FUNCTION_BLOCK FB_IEDServerSession IMPLEMENTS I_ScsmAbortIndEventSink, I_ScsmAssociateIndEventSink, I_ScsmReleaseIndEventSink
VAR_INPUT
	fbConnection		: FB_iec61850ConnectionClass := (ipAbortInd:=THIS^, ipAssociateInd:=THIS^, ipReleaseInd:=THIS^);
END_VAR
VAR
	_bAbort				: BOOL; (* Rising edge activates AbortReq() command execution *)
	_bDisconnect		: BOOL; (* Rising edge activates ReleaseReq() command execution *)
	
	state				: BYTE;
	eState				: E_AsyncEnvironmentState; (* Environment state *)
	bBusy				: BOOL; (* If TRUE => command execution is busy *)
	bSuccess			: BOOL;
	ipResult			: I_AsyncServiceResultClass;
	sLastErrorResult	: T_MaxString;
	fbAbortReason		: FB_ServiceErrorClass := (stError:=SUCCESS_EVENT);
	sLastAbortReason	: T_MaxString;
END_VAR

fbConnection.Execute();
eState:= fbConnection.eState;

(* Execute server control block implementations *)
fbIED.IEDLD1.LLN0.urcb101.Server.Execute();
fbIED.IEDLD1.LLN0.brcb101.Server.Execute();

(* 
	a) The unbuffered report control block IEDLD1/LLN0.urcb101 requires time stamp values in BinaryTime format. 
	We use the unbuffered reporting to test our user defined clock implementation.
	The internal unbuffered report control block implementation queries our user defined clock for new time stamp value.
	
	b) The attribute IEDLD1/MMXU1.TotW.t requires time stamp value in UtcTime format.
	Read of the attribute "IEDLD1/MMXU1.TotW" or "IEDLD1/MMXU1.TotW.t" (e.g. GetDataValues service) triggers the execution IEDLD1/MMXU1.TotW.OnGetVPreEvent() method and 
	queries our user defined clock for new time stamp value.
*)

CASE state OF
	0: (* Initial state *)
		IF _bAbort THEN (* Abort connection => execute AbortReq() command *)
			_bAbort:= FALSE;
			bSuccess:= fbConnection.AbortReq(ipReason:=fbAbortReason, ipSink:=0, ipResult=>ipResult);
			state:= SEL(bSuccess, 100, 1);
		ELSIF eState = E_AsyncEnvironmentState.Established AND _bDisconnect THEN (* Close/release connection => execute ReleaseReq() command *)
			_bDisconnect:= FALSE;
			bSuccess:= fbConnection.ReleaseReq(ipSink:=0, ipResult=>ipResult);
			state:= SEL(bSuccess, 100, 1);
		ELSIF eState = E_AsyncEnvironmentState.Established THEN (* Connection established => exchange IED data *)
			state:= 10;
		END_IF
		_bDisconnect:= FALSE;
		(*==================================================================================================================================================================*)
	1: (* Wait for AbortReq() or ReleaseReq() command completion *)
		IF ipResult <> 0 THEN
			ipResult.Execute();
			IF NOT (bBusy:=ipResult.IsBusy()) THEN
				state:= SEL(ipResult.IsCompleted(), 100(* failed or aborted *), 0(* succeeded *));
			END_IF
		END_IF
		(*==================================================================================================================================================================*)
	10: (* connection established *)
		state:= 0;
		(*==================================================================================================================================================================*)
	100: (* Error state *)
		state:= 0;
		IF ipResult <> 0 THEN
			sLastErrorResult:= ipResult.Dump();
		END_IF
END_CASE

PROPERTY bAbort : BOOL
SET
_bAbort:= bAbort;
END_SET
END_PROPERTY

PROPERTY bDisconnect : BOOL
SET
_bDisconnect:= bDisconnect;
END_SET
END_PROPERTY

(* This method receives IEC61850::Abort.ind primitive. *)
METHOD OnAbortInd
VAR_INPUT
	ipAA		: I_ScsmAssociationClass; (* Application association. If = 0 => optional. *)
	bPAbort		: BOOL; (* TRUE => P-Abort.request(), issued by provider, FALSE => Abort.request(), issued by user. *)
	ipReason	: I_ServiceErrorClass; (* Abort reason. *)
	ipData		: I_BaseStreamClass; (* Optional data. If = 0 => default, no data. *)
END_VAR
VAR
END_VAR
IF ipReason <> 0 THEN
	sLastAbortReason:= ipReason.Dump();
END_IF
END_METHOD

(* This method receives IEC61850::Associate.ind primitive. *)
METHOD OnAssociateInd : BOOL
VAR_INPUT
	ipAA	: I_ScsmAssociationClass; (* Application association. If = 0 => optional. *)
END_VAR
VAR_OUTPUT
	ipResult : I_AsyncServiceResultClass;
END_VAR
VAR
END_VAR
sLastAbortReason:= '';
sLastErrorResult:= '';
OnAssociateInd:= fbConnection.AssociateRsp(ipResult=>ipResult);
END_METHOD

(* This method receives IEC61850::Release.ind primitive. *)
METHOD OnReleaseInd : BOOL
VAR_INPUT
	ipAA	: I_ScsmAssociationClass; (* Application association. If = 0 => optional. *)
END_VAR
VAR_OUTPUT
	ipResult: I_AsyncServiceResultClass;
END_VAR
VAR
END_VAR
OnReleaseInd:= fbConnection.ReleaseRsp(ipResult=>ipResult);
END_METHOD

END_FUNCTION_BLOCK
